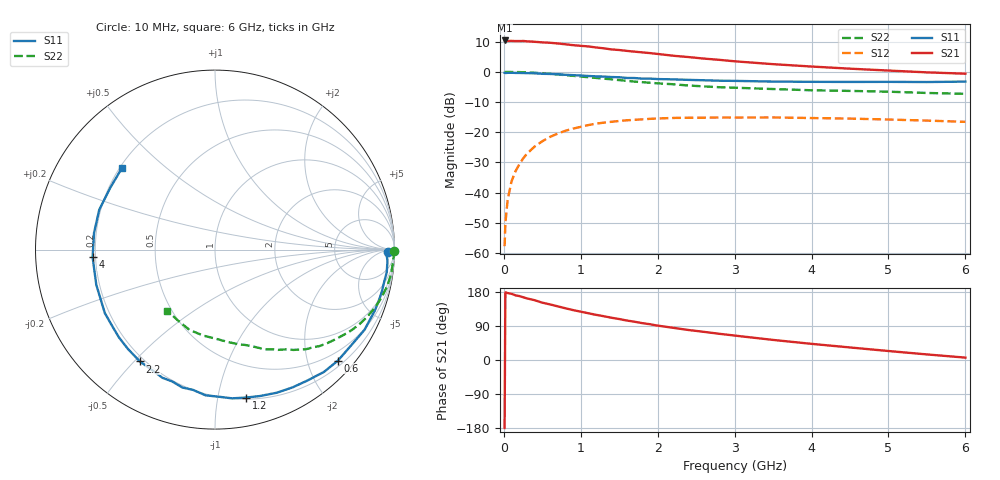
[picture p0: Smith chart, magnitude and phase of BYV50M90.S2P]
! SIEMENS Small Signal Semiconductors
! BFY420
! Si NPN RF SIEGET Grounded Emitter Transistor in MICRO-X
! VCE = 0.5 V  IC = 0.9 mA
! Common Emitter S-Parameters:  October  1996
# GHz  S  MA  R  50
!  f  S11  S21  S12  S22
! GHz  MAG  ANG  MAG  ANG  MAG  ANG  MAG  ANG
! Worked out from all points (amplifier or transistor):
!   36 points, 10 MHz to 6 GHz, reference 50 ohm
!   highest |S21| = 10.4 dB at 10 MHz (marker M1)
!   |S21| within 3 dB of that: start of sweep to 1.415 GHz
!   unconditionally stable (mu >= 1): 4.565 GHz to end of sweep
!   at 250 MHz: K = 0.03, MSG = 19.5 dB, |S12| = -28.7 dB
!   at 1.4 GHz: K = 0.26, MSG = 12.0 dB, |S12| = -16.5 dB
!   at 6 GHz: K = 1.34, MAG = 4.5 dB, |S12| = -16.6 dB
!   S11 on the Smith chart (normalised r, x): 10 MHz: 46, -19; 600 MHz: 0.31, -2.57; 1.2 GHz: 0.21, -1.21; 2.2 GHz: 0.18, -0.52; 4 GHz: 0.19, -0.03; 6 GHz: 0.21, +0.36
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0.01  0.9634 -0.9  3.307 -179.4  0.0013 92.9  0.9968 -0.4
0.02  0.9562 -1.6  3.283 178.7  0.0031 93.6  0.9953 -0.8
0.05  0.9629 -3.7  3.233 176.6  0.0077 87.2  0.9963 -2.0
0.1  0.9653 -7.5  3.255 174.7  0.0154 85.8  0.9937 -4.2
0.15  0.9597 -10.7  3.226 170.7  0.0224 82.0  0.9916 -6.3
0.2  0.9586 -14.3  3.23 168.8  0.0293 81.2  0.9898 -8.2
0.25  0.9557 -17.8  3.241 165.6  0.0367 78.5  0.9844 -10.4
0.3  0.9528 -21.0  3.202 162.6  0.0442 76.4  0.9794 -12.4
0.5  0.9274 -35.2  3.072 151.3  0.0709 67.2  0.9467 -20.2
0.6  0.9228 -42.1  3.029 146.7  0.0838 62.8  0.9265 -23.9
0.8  0.8928 -54.8  2.855 136.5  0.1057 54.4  0.8819 -30.8
1.1  0.8535 -72.9  2.632 123.3  0.1316 43.5  0.8142 -39.8
1.2  0.8423 -78.2  2.531 119.1  0.1387 40.1  0.7926 -42.7
1.6  0.7912 -98.9  2.222 104.1  0.1577 28.6  0.7094 -52.0
2  0.7588 -116.7  1.977 90.7  0.1689 19.3  0.6448 -59.5
2.2  0.7506 -123.9  1.848 85.0  0.1725 15.0  0.6231 -63.2
2.8  0.7127 -144.1  1.58 69.2  0.1754 5.3  0.5565 -72.6
3.5  0.6898 -163.5  1.34 53.0  0.1758 -3.2  0.519 -82.2
4  0.6832 -176.4  1.224 42.6  0.1719 -8.4  0.4952 -90.1
4.5  0.6803 172.1  1.128 33.1  0.1682 -13.2  0.4833 -98.0
5.5  0.6778 149.3  0.98 14.7  0.1559 -19.7  0.4469 -117.0
6  0.6889 139.0  0.931 6.3  0.1487 -20.8  0.4323 -127.8
